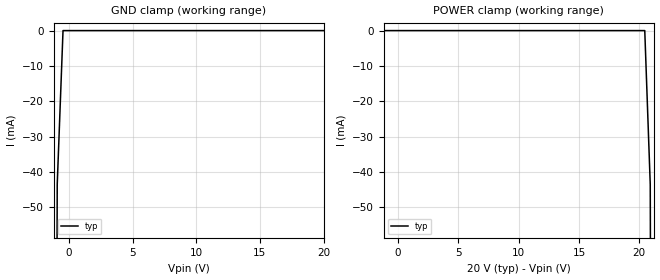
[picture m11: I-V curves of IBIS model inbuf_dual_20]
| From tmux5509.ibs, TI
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| inbuf_dual_20
[Model]   inbuf_dual_20
Model_type   Input
Vinl = 0.7
Vinh = 1.2
|   typ   min   max
C_comp   1.008417e-12   NA   NA
[Voltage Range]   20   NA   NA
[Temperature Range]   27   NA   NA
[Power Clamp Reference]   20   NA   NA
[GND Clamp Reference]   0   NA   NA
[GND Clamp]
|   Voltage   I(typ)   I(min)   I(max)
-25V      -45.95A    NA         NA
-1.364V   -576mA     NA         NA
-909.1mV  -43.46mA   NA         NA
-454.5mV  -746nA     NA         NA
20V       326.5nA    NA         NA
[POWER Clamp]
|   Voltage   I(typ)   I(min)   I(max)
-5V       818.1nA    NA         NA
20.45V    -746nA     NA         NA
20.91V    -43.46mA   NA         NA
21.36V    -576mA     NA         NA
40V       -31.07A    NA         NA
